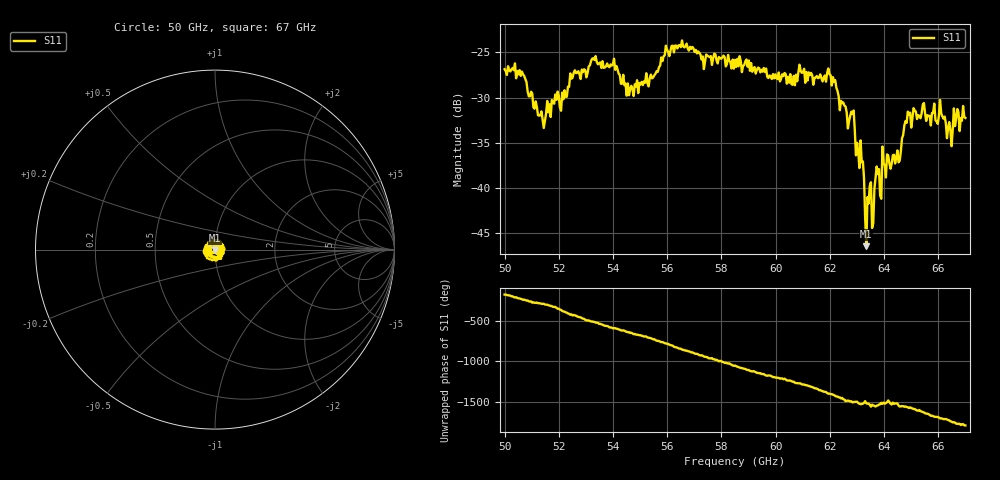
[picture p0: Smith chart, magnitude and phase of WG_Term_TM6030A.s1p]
!Agilent Technologies,E8361A,US42410132,A.06.03.05
!Agilent E8361A: A.06.03.05
!Date: Friday, July 11, 2008 15:41:04
!Correction: S11(Full 2 Port(1,2))
!S1P File: Measurement: S11:
# Hz S  MA  R 50
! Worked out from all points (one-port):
!   401 points, 50 GHz to 67 GHz, reference 50 ohm
!   lowest |S11| = -46.5 dB at 63.34 GHz (marker M1), VSWR 1.01, Z = 50.1 - j0.469 ohm
!   |S11| at or under -10 dB: start of sweep to end of sweep
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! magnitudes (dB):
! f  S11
! 50 GHz  -26.9
! 50.64 GHz  -27.1
! 51.4 GHz  -32.4
! 52.12 GHz  -29.5
! 52.51 GHz  -27.8
! 53.27 GHz  -25.6
! 54.25 GHz  -27.5
! 54.67 GHz  -28.7
! 56.38 GHz  -24.6
! 58.5 GHz  -25.8
! 60.62 GHz  -28.6
! 60.97 GHz  -27.3
! 61.94 GHz  -26.8
! 62.75 GHz  -32.0
! 62.84 GHz  -31.8
! 63.01 GHz  -35.0
! 63.17 GHz  -37.2
! 63.34 GHz  -46.5
! 63.6 GHz  -43.9
! 63.73 GHz  -37.6
! 63.81 GHz  -37.9
! 64.03 GHz  -37.5
! 64.53 GHz  -37.2
! 64.88 GHz  -31.6
! 66.15 GHz  -32.1
! 66.41 GHz  -32.7
! 66.66 GHz  -32.3
! 67 GHz  -32.3
